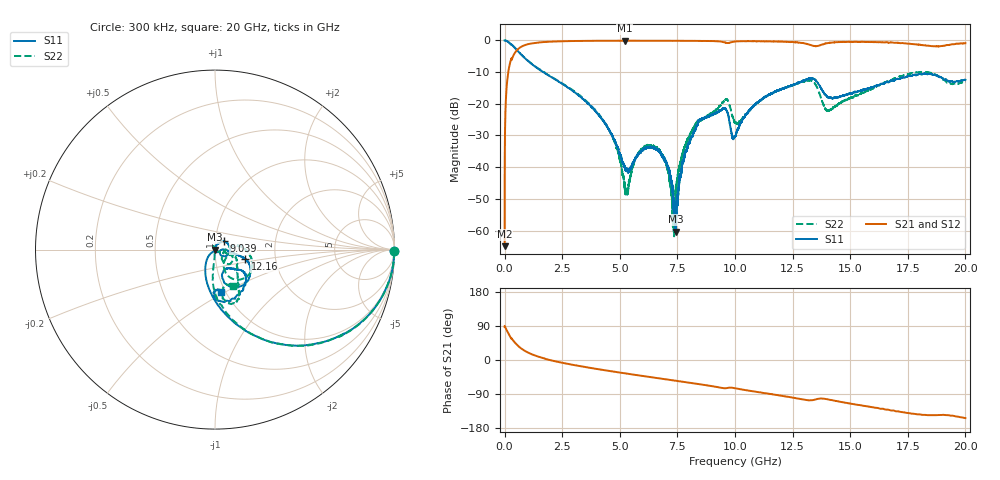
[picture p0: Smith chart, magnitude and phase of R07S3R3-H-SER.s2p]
!{R07S3R3}
!Johanson Technology Inc.
!www.johansontechnology.com
!Test Board Conditions:
!Substrate Type  RO4350B
!Substrate Thickness  10 mil
!Substrate Dk  3.66
!TL Type: GCPW
!TL Trace Width  21 mil
!TL Gap  20 mil
!Electrode orientation  Horizontal
!DUT TOPOLOGY	SERIES
!Mounting Pad LxW  16x21 mil
! Created Sat Feb  6 11:30:52 2021
# hz S ma R 50
! 2 Port Network Data from SP1.SP block
! freq  magS11  angS11  magS21  angS21  magS12  angS12  magS22  angS22
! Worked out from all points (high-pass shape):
!   20001 points, 300 kHz to 20 GHz, reference 50 ohm
!   highest |S21| = -0.07 dB at 5.213 GHz (marker M1); lowest = -64.9 dB at 300 kHz (marker M2)
!   |S21| within 3 dB of the highest: 535.6 MHz to end of sweep
!   lowest |S11| = -60.3 dB at 7.42 GHz (marker M3), VSWR 1.00, Z = 49.9 - j0.0701 ohm
!   |S11| at or under -10 dB: 1.677 GHz to end of sweep
!   |S22| runs from -61.8 to 0.0 dB; largest |S21 - S12| = 0.012
!   S11 on the Smith chart (normalised r, x): 300 kHz: open; 9.039 GHz: 1.10, +0.10; 12.16 GHz: 1.40, -0.15; 20 GHz: 0.95, -0.48
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300000  1 -0.4  0.0005658 87.5  0.0006617 92.5  0.9998 -0.5
1.183e8  0.9694 -15.1  0.2401 75.2  0.2403 75.2  0.97 -15.1
3.673e8  0.8193 -37.7  0.5636 51.7  0.5644 51.8  0.8195 -37.7
1.2503e9  0.4051 -76.6  0.9078 13.4  0.9072 13.4  0.4092 -75.4
3.3343e9  0.1253 -115.7  0.9843 -16.8  0.984 -16.8  0.1289 -95.2
4.6013e9  0.03486 -137.8  0.9895 -29.4  0.99 -29.4  0.03437 -93.5
5.2133e9  0.01039 -107.9  0.9916 -35.1  0.9909 -35.1  0.005361 -122.7
5.8953e9  0.01708 -38.1  0.9897 -41.3  0.9901 -41.3  0.01792 116.2
6.6673e9  0.01871 -53.7  0.9894 -48.1  0.989 -48.1  0.01874 121.1
7.0523e9  0.01079 -68.4  0.9879 -51.4  0.9879 -51.5  0.01035 121.6
7.3093e9  0.003761 -97.2  0.9877 -53.7  0.9883 -53.7  0.001167 64.9
7.4203e9  0.0009639 -133.2  0.9869 -54.7  0.9875 -54.7  0.003689 -20.3
7.8953e9  0.018 83.6  0.9858 -58.9  0.9859 -58.9  0.02502 -27.7
8.4603e9  0.05584 50.6  0.983 -63.9  0.982 -64.0  0.05362 -10.9
9.0393e9  0.06659 43.4  0.9776 -69.4  0.977 -69.5  0.07357 -18.2
9.6223e9  0.07993 -17.0  0.9179 -74.4  0.9179 -74.3  0.117 -37.5
1.00003e10  0.03017 -7.7  0.9632 -74.5  0.9619 -74.6  0.04949 -38.3
1.21643e10  0.1779 -17.5  0.9523 -95.8  0.9505 -95.8  0.1778 -3.1
1.33343e10  0.2531 -50.7  0.8343 -106.1  0.8346 -106.2  0.2305 -42.8
1.40503e10  0.126 -67.9  0.9102 -104.1  0.9093 -104.2  0.07752 -36.0
1.66673e10  0.2194 -39.8  0.922 -131.2  0.9265 -131.7  0.2309 -55.6
2e10  0.2395 -82.1  0.9058 -153.3  0.9018 -153.2  0.2258 -63.9
